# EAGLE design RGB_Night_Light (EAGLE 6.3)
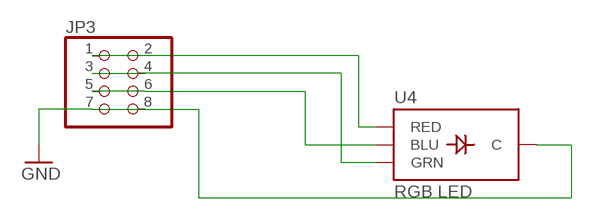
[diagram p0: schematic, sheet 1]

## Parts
JP3  PINHD-2X4  [2X04]
U4  RGB LED  LED-TRICOLOR-THROUGHHOLE  [LED-TRICOLOR-THROUGHHOLE]

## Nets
GND: JP3.7 JP3.8 U4.GND(C)
N$15: JP3.1 JP3.2 U4.RED
N$24: JP3.5 JP3.6 U4.BLU
N$25: JP3.3 JP3.4 U4.GRN

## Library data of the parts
JP3 = adafruit:PINHD-2X4: PIN HEADER
U4 = E-Paper Display 2:LED-TRICOLOR-THROUGHHOLE

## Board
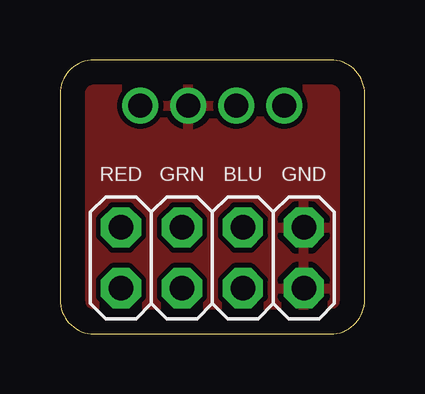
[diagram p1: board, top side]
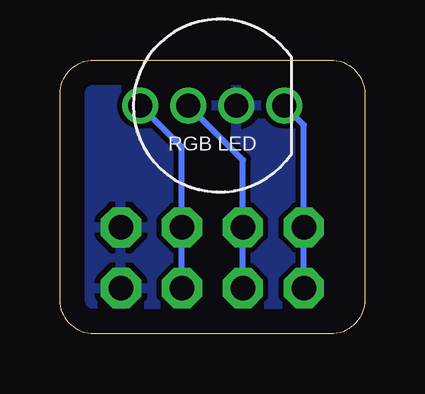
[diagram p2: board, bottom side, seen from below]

Size 12.7 x 11.43 mm. Coordinates in mm from the lower left corner, seen from the top.
Outline: 1.42,0 11.28,0 arc90 12.7,1.42 12.7,10.01 arc90 11.28,11.43 1.42,11.43 arc90 0,10.01 0,1.42 arc90 1.42,0
Copper layers (1*16): Top 0.035mm / dielectric 1.5mm / Bottom 0.035mm
Design rules "default": minimum track width 10mil, minimum drill 24mil, track to track 8mil, track to pad 8mil, pad to pad 8mil, via to via 8mil, smd to smd 8mil, copper to edge 40mil, drill to drill 8mil, minimum pad ring 10mil, minimum via ring 8mil, stop-mask expansion 4mil, vias tented up to drill 0mil, thermal gap 10mil

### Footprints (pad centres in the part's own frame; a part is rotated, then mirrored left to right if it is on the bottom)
2X04 = drill 1.016 pad 1.676 octagon: 1 -3.81,-1.27; 2 -3.81,1.27; 3 -1.27,-1.27; 4 -1.27,1.27; 5 1.27,-1.27; 6 1.27,1.27; 7 3.81,-1.27; 8 3.81,1.27
LED-TRICOLOR-THROUGHHOLE = drill 1: BLU 3,0; GND -1,0; GRN 1,0; RED -3,0

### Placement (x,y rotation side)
JP3  6.35,3.17 0 top
U4  6.35,9.52 180 bottom

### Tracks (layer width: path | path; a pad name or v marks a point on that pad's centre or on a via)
GND
  pour Top: -1.27,13.34 13.97,13.34 13.97,-0.64 -1.27,-0.64
  pour Bottom: -1.27,13.34 13.97,13.34 13.97,-0.64 -1.27,-0.64
N$15
  Bottom 0.254: U4.RED 2.54,8.71 JP3.2 JP3.1
N$24
  Bottom 0.254: JP3.5 JP3.6 7.62,7.79 U4.BLU
N$25
  Bottom 0.254: JP3.3 JP3.4 5.08,7.25 U4.GRN

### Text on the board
tNames: RED | GRN | BLU | GND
